| This Model is valid for Temperature Range -40C<=Tc<=95C
| Valid for DDR4-2666/3200 operation
| Part Number   VDD/VDDQ   Architecture   Package
| SCB12Q4G160BF   1.20V/1.20V   256Mx16   BGA96
[IBIS ver] 5.1
[File name]  usssq4g16bi.ibs
[File Rev]  1.0
[Date]   2024-06-12
[Notes]   IBIS Model Revision History
   Rev 1.0 : 2024-06-12, Initial release
[Source]   Simulation of a silicon level SPICE model
[Disclaimer]  The IBIS models are for modeling purpose only and are
   subject to change without any notice. UniIC is not
   responsible for any problems the models may cause.
[Copyright]   Copyright 2024 UniIC Semiconductors Corp. All rights reserved
|   Component : SCB12Q4G160BF (BGA96 X16)
[Component] SCB12Q4G160BF
[Manufacturer] UniIC Semiconductors Corp.
[Package]
| variable   typ   min   max
R_pkg   0.000E+00   0.000E+00   1.504E+00
L_pkg   0.000E+00   0.000E+00   3.900E-09
C_pkg   0.000E+00   0.000E+00   0.860E-12
[Pin]  signal_name   model_name   R_pin   L_pin   C_pin
A1   VDDQ   POWER
A2   VSS   GND
A3   DQU0   DQ   1.061E+00 1.816E-09 0.604E-12
A7   DQSU_C   DQS   1.097E+00 1.932E-09 0.627E-12
A8   VSS   GND
A9   VDDQ   POWER
B1   VPP   POWER
B2   VSS   GND
B3   VDD   POWER
B7   DQSU_T   DQS   1.086E+00 1.895E-09 0.635E-12
B8   DQU1   DQ   1.060E+00 1.678E-09 0.635E-12
B9   VDD   POWER
C1   VDDQ   POWER
C2   DQU4   DQ   1.005E+00 1.541E-09 0.595E-12
C3   DQU2   DQ   0.978E+00 1.760E-09 0.579E-12
C7   DQU3   DQ   0.997E+00 1.651E-09 0.603E-12
C8   DQU5   DQ   0.996E+00 1.573E-09 0.599E-12
C9   VSS   GND
D1   VDD   POWER
D2   VSS   GND
D3   DQU6   DQ   0.998E+00 1.596E-09 0.598E-12
D7   DQU7   DQ   0.966E+00 1.587E-09 0.591E-12
D8   VSS   GND
D9   VDDQ   POWER
E1   VSS   GND
E2   DMU_N   DM   0.999E+00 1.658E-09 0.571E-12
E3   VSS   GND
E7   DML_N   DM   0.726E+00 1.206E-09 0.454E-12
E8   VSS   GND
E9   VSS   GND
F1   VSS   GND
F2   VDDQ   POWER
F3   DQSL_C   DQS   0.723E+00 1.349E-09 0.447E-12
F7   DQL1   DQ   0.736E+00 1.249E-09 0.454E-12
F8   VDDQ   POWER
F9   ZQ   NC
G1   VDDQ   POWER
G2   DQL0   DQ   0.714E+00 1.214E-09 0.441E-12
G3   DQSL_T   DQS   0.720E+00 1.356E-09 0.447E-12
G7   VDD   POWER
G8   VSS   GND
G9   VDDQ   POWER
H1   VSS   GND
H2   DQL4   DQ   0.736E+00 1.295E-09 0.454E-12
H3   DQL2   DQ   0.707E+00 1.305E-09 0.441E-12
H7   DQL3   DQ   0.739E+00 1.221E-09 0.454E-12
H8   DQL5   DQ   0.745E+00 1.177E-09 0.469E-12
H9   VSS   GND
J1   VDD   POWER
J2   VDDQ   POWER
J3   DQL6   DQ   0.712E+00 1.299E-09 0.441E-12
J7   DQL7   DQ   0.753E+00 1.231E-09 0.467E-12
J8   VDDQ   POWER
J9   VDD   POWER
K1   VSS   GND
K2   CKE   CA   0.839E+00 1.833E-09 0.610E-12
K3   ODT   CA   0.814E+00 1.650E-09 0.604E-12
K7   CK_T   CK   1.190E+00 2.399E-09 0.655E-12
K8   CK_C   CK   1.097E+00 2.649E-09 0.501E-12
K9   VSS   GND
L1   VDD   POWER
L2   WE_N   CA   1.069E+00 2.315E-09 0.563E-12
L3   ACT_N   CA   0.965E+00 1.945E-09 0.687E-12
L7   CS_N   CA   0.802E+00 1.763E-09 0.601E-12
L8   RAS_N   CA   0.802E+00 1.763E-09 0.601E-12
L9   VDD   POWER
M1   VREFCA   POWER   0.802E+00 1.763E-09 0.601E-12
M2   BG0   CA   0.802E+00 1.763E-09 0.601E-12
M3   A10   CA   0.802E+00 1.763E-09 0.601E-12
M7   A12   CA   0.802E+00 1.763E-09 0.601E-12
M8   CAS_N   CA   0.802E+00 1.763E-09 0.601E-12
M9   VSS   GND
N1   VSS   GND
N2   BA0   CA   1.024E+00 2.812E-09 0.573E-12
N3   A4   CA   1.165E+00 3.254E-09 0.572E-12
N7   A3   CA   1.172E+00 3.162E-09 0.563E-12
N8   BA1   CA   1.034E+00 2.774E-09 0.614E-12
N9   TEN   TEN   0.802E+00 2.106E-09 0.743E-12
P1   RESET_N   RST   1.049E+00 1.763E-09 0.601E-12
P2   A6   CA   1.249E+00 3.308E-09 0.699E-12
P3   A0   CA   1.215E+00 3.266E-09 0.630E-12
P7   A1   CA   1.245E+00 3.351E-09 0.652E-12
P8   A5   CA   1.307E+00 3.330E-09 0.717E-12
P9   ALERT_N   ALE   1.273E+00 2.542E-09 0.863E-12
R1   VDD   POWER
R2   A8   CA   1.261E+00 3.323E-09 0.696E-12
R3   A2   CA   1.300E+00 3.266E-09 0.731E-12
R7   A9   CA   1.365E+00 2.951E-09 0.708E-12
R8   A7   CA   1.261E+00 3.322E-09 0.703E-12
R9   VPP   POWER
T1   VSS   GND
T2   A11   CA   1.504E+00 3.733E-09 0.825E-12
T3   PAR   CA   1.383E+00 3.131E-09 0.756E-12
T7   NC   NC
T8   A13   CA   1.476E+00 3.690E-09 0.806E-12
T9   VDD   POWER
[Pin Mapping]  pulldown_ref   pullup_ref   gnd_clamp_ref   power_clamp_ref   ext_ref
A1   NC   VDDQ
A2   VSS   NC
A3   VSS   VDDQ   VSS   VDDQ
A7   VSS   VDDQ   VSS   VDDQ
A8   VSS   NC
A9   NC   VDDQ
B1   NC   VPP
B2   VSS   NC
B3   NC   VDD
B7   VSS   VDDQ   VSS   VDDQ
B8   VSS   VDDQ   VSS   VDDQ
B9   NC   VDD
C1   NC   VDDQ
C2   VSS   VDDQ   VSS   VDDQ
C3   VSS   VDDQ   VSS   VDDQ
C7   VSS   VDDQ   VSS   VDDQ
C8   VSS   VDDQ   VSS   VDDQ
C9   VSS   NC
D1   NC   VDD
D2   VSS   NC
D3   VSS   VDDQ   VSS   VDDQ
D7   VSS   VDDQ   VSS   VDDQ
D8   VSS   NC
D9   NC   VDDQ
E1   VSS   NC
E2   VSS   VDDQ   VSS   VDDQ
E3   VSS   NC
E7   VSS   VDDQ   VSS   VDDQ
E8   VSS   NC
E9   VSS   NC
F1   VSS   NC
F2   NC   VDDQ
F3   VSS   VDDQ   VSS   VDDQ
F7   VSS   VDDQ   VSS   VDDQ
F8   NC   VDDQ
F9   NC   NC
G1   NC   VDDQ
G2   VSS   VDDQ   VSS   VDDQ
G3   VSS   VDDQ   VSS   VDDQ
G7   NC   VDD
G8   VSS   NC
G9   NC   VDDQ
H1   VSS   NC
H2   VSS   VDDQ   VSS   VDDQ
H3   VSS   VDDQ   VSS   VDDQ
H7   VSS   VDDQ   VSS   VDDQ
H8   VSS   VDDQ   VSS   VDDQ
H9   VSS   NC
J1   NC   VDD
J2   NC   VDDQ
J3   VSS   VDDQ   VSS   VDDQ
J7   VSS   VDDQ   VSS   VDDQ
J8   NC   VDDQ
J9   NC   VDD
K1   VSS   NC
K2   NC   NC   VSS   VDD
K3   NC   NC   VSS   VDD
K7   NC   NC   VSS   VDD
K8   NC   NC   VSS   VDD
K9   VSS   NC
L1   NC   VDD
L2   NC   NC   VSS   VDD
L3   NC   NC   VSS   VDD
L7   NC   NC   VSS   VDD
L8   NC   NC   VSS   VDD
L9   NC   VDD
M1   NC   VREFCA
M2   NC   NC   VSS   VDD
M3   NC   NC   VSS   VDD
M7   NC   NC   VSS   VDD
M8   NC   NC   VSS   VDD
M9   VSS   NC
N1   VSS   NC
N2   NC   NC   VSS   VDD
N3   NC   NC   VSS   VDD
N7   NC   NC   VSS   VDD
N8   NC   NC   VSS   VDD
N9   NC   NC   VSS   VDD
P1   NC   NC   VSS   VDD
P2   NC   NC   VSS   VDD
P3   NC   NC   VSS   VDD
P7   NC   NC   VSS   VDD
P8   NC   NC   VSS   VDD
P9   VSS   VDD   VSS   VDD
R1   NC   VDD
R2   NC   NC   VSS   VDD
R3   NC   NC   VSS   VDD
R7   NC   NC   VSS   VDD
R8   NC   NC   VSS   VDD
R9   NC   VPP
T1   VSS   NC
T2   NC   NC   VSS   VDD
T3   NC   NC   VSS   VDD
T7   NC   NC
T8   NC   NC   VSS   VDD
T9   NC   VDD
[Diff pin]  inv_pin  vdiff   tdelay_typ   tdelay_min   tdelay_max
B7   A7   1.400E-01  NA   NA   0.000E+00
G3   F3   1.400E-01  NA   NA   0.000E+00
K7   K8   1.800E-01  NA   NA   0.000E+00
[Model Selector] DQ
DQ_34 34 Ohm Data I/O with no ODT
DQ_48 48 Ohm Data I/O with no ODT
DQ_ODT_34 Data Input with 34 Ohm ODT
DQ_ODT_40 Data Input with 40 Ohm ODT
DQ_ODT_48 Data Input with 48 Ohm ODT
DQ_ODT_60 Data Input with 60 Ohm ODT
DQ_ODT_80 Data Input with 80 Ohm ODT
DQ_ODT_120 Data Input with 120 Ohm ODT
DQ_ODT_240 Data Input with 240 Ohm ODT
DQ_RCV Data Input with no ODT
[Model Selector] DQS
DQS_34 34 Ohm Data Strobe I/O with no ODT
DQS_48 48 Ohm Data Strobe I/O with no ODT
DQS_ODT_34 Data Strobe Input with 34 Ohm ODT
DQS_ODT_40 Data Strobe Input with 40 Ohm ODT
DQS_ODT_48 Data Strobe Input with 48 Ohm ODT
DQS_ODT_60 Data Strobe Input with 60 Ohm ODT
DQS_ODT_80 Data Strobe Input with 80 Ohm ODT
DQS_ODT_120 Data Strobe Input with 120 Ohm ODT
DQS_ODT_240 Data Strobe Input with 240 Ohm ODT
DQS_RCV Data Strobe Input with no ODT
[Model Selector] DM
DQ_34 34 Ohm Data I/O with no ODT
DQ_48 48 Ohm Data I/O with no ODT
DQ_ODT_34 Data Input with 34 Ohm ODT
DQ_ODT_40 Data Input with 40 Ohm ODT
DQ_ODT_48 Data Input with 48 Ohm ODT
DQ_ODT_60 Data Input with 60 Ohm ODT
DQ_ODT_80 Data Input with 80 Ohm ODT
DQ_ODT_120 Data Input with 120 Ohm ODT
DQ_ODT_240 Data Input with 240 Ohm ODT
DQ_RCV Data Input with no ODT
[Model Selector] ALE
ALE_DRV ALERT_N Data I/O with no ODT
ALE_RCV Data Input with no ODT
| Models and submodels in the file (26): DQ_34 (I/O), DQ_48 (I/O), DQ_ODT_34 (Input), DQ_ODT_40 (Input), DQ_ODT_48 (Input), DQ_ODT_60 (Input), DQ_ODT_80 (Input), DQ_ODT_120 (Input), DQ_ODT_240 (Input), DQ_RCV (Input), DQS_34 (I/O), DQS_48 (I/O), DQS_ODT_34 (Input), DQS_ODT_40 (Input), DQS_ODT_48 (Input), DQS_ODT_60 (Input), DQS_ODT_80 (Input), DQS_ODT_120 (Input), DQS_ODT_240 (Input), DQS_RCV (Input), ALE_DRV (Open_sink), ALE_RCV (Input), CA (Input), CK (Input), RST (Input), TEN (Input)
